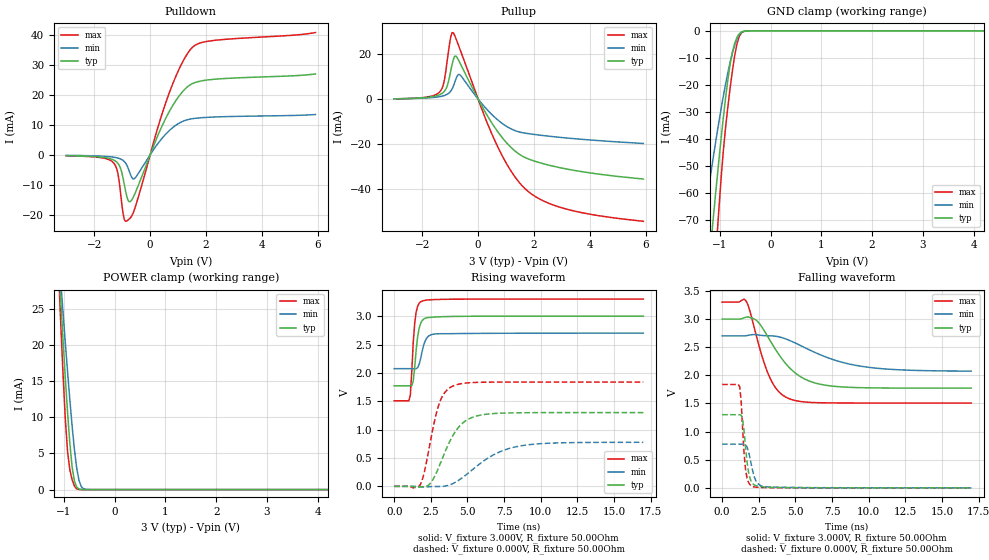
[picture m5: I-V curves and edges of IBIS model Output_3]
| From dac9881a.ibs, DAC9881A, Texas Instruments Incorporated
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|   Output_3 MODEL
[Model]   Output_3
Model_type   3-state
| Signals
Cref  = 4.5pF   |Timing specification test load capacitance value
Rref  = 5000Ohm
Vref  = 2.5V
Vmeas = 1.5V
| variable   typ   min   max
|Output tri-stated
C_comp   3.676pF   4.331pF   2.899pF
|Output high
|C_comp   6.262pF   7.145pF   5.319pF
|Output low
|C_comp   6.894pF   7.074pF   5.827pF
[Voltage Range]   3.000V   2.700V   3.300V
| Junction Temperature (Ambient temp is 25C typ, 105C min,  -40C max)
[Temperature Range]   27.0   105.0   -40.0
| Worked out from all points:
|   slope of the pulldown table from 0 to 0.45 V, typ, clamps not added: 44.4 ohm
|   slope of the pullup table from 0 to 0.45 V, typ, clamps not added: 46 ohm
|   GND clamp passes 1 mA (typ) near -0.61 V on its own axis
|   POWER clamp passes 1 mA (typ) near -0.78 V on its own axis
|   falling waveform, V_fixture 3.000V, R_fixture 50.00Ohm: 20-80 % time 2.15ns typ, 3.72ns min, 1.34ns max; typ from 3 V to 1.77 V
|   rising waveform, V_fixture 3.000V, R_fixture 50.00Ohm: 20-80 % time 313ps typ, 388ps min, 271ps max; typ from 1.77 V to 3 V
|   rising waveform, V_fixture 0.000V, R_fixture 50.00Ohm: 20-80 % time 1.48ns typ, 2.66ns min, 936ps max; typ from 0 V to 1.3 V
|   falling waveform, V_fixture 0.000V, R_fixture 50.00Ohm: 20-80 % time 335ps typ, 436ps min, 270ps max; typ from 1.3 V to 0 V
[Pulldown]
|   Voltage   I(typ)   I(min)   I(max)
-3V       -315.2uA   -207.5uA   -347.1uA
-1.335V   -1.633mA   -781.9uA   -2.46mA
-1.155V   -2.871mA   -1.108mA   -6.189mA
-1.065V   -4.405mA   -1.394mA   -12.3mA
-930mV    -9.697mA   -2.211mA   -21.49mA
-840mV    -13.8mA    -3.377mA   -22.14mA
-750mV    -15.73mA   -5.432mA   -21.48mA
-570mV    -13.51mA   -8.027mA   -18.49mA
600mV     12.98mA    7.307mA    18.53mA
1.095V    20.36mA    10.86mA    29.8mA
1.5V      23.72mA    12.03mA    35.79mA
5.91V     26.98mA    13.44mA    40.82mA
[GND Clamp]
|   Voltage   I(typ)   I(min)   I(max)
-3V       -500.5mA   -338.5mA   -693.5mA
-1.335V   -112.2mA   -73.35mA   -160.5mA
-1.29V    -102.6mA   -67.34mA   -146.6mA
-1.155V   -74.56mA   -50.01mA   -105.4mA
-1.11V    -65.55mA   -44.49mA   -92.01mA
-1.065V   -56.74mA   -39.13mA   -78.97mA
-1.02V    -48.18mA   -33.92mA   -66.43mA
-930mV    -32.01mA   -24.1mA    -44.24mA
-795mV    -12.16mA   -11.45mA   -20.92mA
-660mV    -2.339mA   -2.894mA   -4.688mA
-570mV    -387.6uA   -568.8uA   -684.4uA
5.91V     0A         0A         0A
[Pullup]
|   Voltage   I(typ)   I(min)   I(max)
-3V       90.07uA    84.6uA     74.35uA
-1.38V    1.871mA    1.036mA    3.061mA
-1.245V   2.905mA    1.401mA    6.232mA
-1.11V    5.586mA    2.059mA    16.47mA
-975mV    12.63mA    3.53mA     27.63mA
-885mV    17.54mA    5.673mA    29.29mA
-660mV    16.21mA    10.82mA    22.41mA
600mV     -12.64mA   -8.121mA   -18.44mA
1.14V     -20.96mA   -12.96mA   -31.12mA
1.68V     -25.89mA   -15.09mA   -39.68mA
3.12V     -30.85mA   -17.18mA   -48.56mA
5.91V     -35.4mA    -19.66mA   -54.09mA
[POWER Clamp]
|   Voltage   I(typ)   I(min)   I(max)
-3V       213.2mA    183.1mA    247.3mA
-1.11V    32.27mA    33.32mA    30.73mA
-1.065V   26.47mA    28.94mA    23.24mA
-1.02V    20.89mA    24.65mA    16.18mA
-975mV    15.61mA    20.46mA    9.948mA
-930mV    10.74mA    16.38mA    5.304mA
-885mV    6.457mA    12.47mA    2.746mA
-840mV    3.156mA    8.831mA    1.373mA
-750mV    359.7uA    3.01mA     107.9uA
-660mV    18uA       424.2uA    3.017uA
-525mV    211.4nA    8.261uA    20.67nA
5.91V     0A         0A         0A
[Ramp]
R_load = 50.00Ohm
|   typ   min   max
dV/dt_r   779.958mV/1.475ns   465.797mV/2.661ns   1.103V/936.338ps
dV/dt_f   736.722mV/2.148ns   375.476mV/3.716ns   1.076V/1.336ns
[Falling Waveform]
V_fixture = 3.000V
V_fixture_min = 2.700V
V_fixture_max = 3.300V
R_fixture = 50.00Ohm
|   Time   V(typ)   V(min)   V(max)
0s        3V         2.7V       3.3V
1.6ns     3.03V      2.702V     3.332V
1.9ns     3.026V     2.717V     3.138V
2.4ns     2.962V     2.72V      2.637V
3.2ns     2.65V      2.702V     1.991V
3.8ns     2.397V     2.688V     1.728V
4.6ns     2.133V     2.619V     1.582V
6.3ns     1.867V     2.41V      1.516V
9.4ns     1.781V     2.164V     1.508V
17ns      1.772V     2.074V     1.507V
[Rising Waveform]
V_fixture = 3.000V
V_fixture_min = 2.700V
V_fixture_max = 3.300V
R_fixture = 50.00Ohm
|   Time   V(typ)   V(min)   V(max)
0s        1.772V     2.074V     1.507V
1ns       1.772V     2.074V     1.507V
1.1ns     1.772V     2.074V     1.607V
1.3ns     1.859V     2.074V     2.536V
1.4ns     2.097V     2.074V     2.879V
1.6ns     2.638V     2.092V     3.175V
1.9ns     2.919V     2.372V     3.265V
2.2ns     2.97V      2.606V     3.283V
2.8ns     2.985V     2.686V     3.293V
17ns      3V         2.7V       3.3V
[Rising Waveform]
V_fixture = 0.000V
V_fixture_min = 0.000V
V_fixture_max = 0.000V
R_fixture = 50.00Ohm
|   Time   V(typ)   V(min)   V(max)
0s        4.326uV    19.91uV    -6.686uV
1.8ns     -10.46mV   -8.785mV   38.11mV
2ns       -6.66mV    -15.73mV   191.7mV
2.4ns     34.49mV    -6.467mV   695.2mV
3ns       311.8mV    -2.758mV   1.401V
3.4ns     564.6mV    2.208mV    1.635V
4ns       893.9mV    48.67mV    1.767V
5.4ns     1.222V     306.8mV    1.83V
8.3ns     1.296V     696.8mV    1.838V
17ns      1.3V       776.3mV    1.838V
[Falling Waveform]
V_fixture = 0.000V
V_fixture_min = 0.000V
V_fixture_max = 0.000V
R_fixture = 50.00Ohm
|   Time   V(typ)   V(min)   V(max)
0s        1.3V       776.3mV    1.838V
1.2ns     1.3V       776.1mV    1.795V
1.3ns     1.294V     776.1mV    1.541V
1.4ns     1.213V     776.8mV    1.042V
1.6ns     724.9mV    770.6mV    325.3mV
1.8ns     281.6mV    646.4mV    96.58mV
2.1ns     70.6mV     285.3mV    21.68mV
2.4ns     32.34mV    87.53mV    10.95mV
3.1ns     11.92mV    17.74mV    4.766mV
17ns      4.326uV    19.91uV    -6.686uV
